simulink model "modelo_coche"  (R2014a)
settings: Solver=ode23t  StartTime=0.0  StopTime=10.0  MaxStep=0.2  RelTol=1e-3
undefined symbols (not defined in the file): inertiaLateral
libraries: nesl_utility x18, fl_lib x18, sdl_lib x10, simulink x1

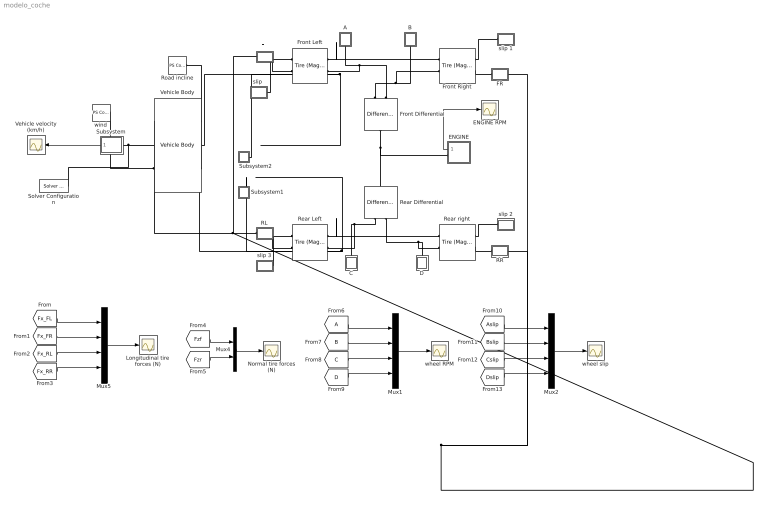
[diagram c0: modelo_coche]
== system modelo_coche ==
  A : Subsystem
  B : Subsystem
  C : Subsystem
  D : Subsystem
  ENGINE : Subsystem
  ENGINE RPM : Scope
  FL : Subsystem
  FR : Subsystem
  From6 : From  TagVisibility=global
  Front Differential : sdl_lib/Gears/Differential  driveshaft_location=2  cd_ratio=4  friction_model=1  efficiency=[ 0.85 0.92 ]  mu_visc=[ 0 0 ] N*m/(rad/s)  w_thr=[ 0.01 0.01 ] rad/s
  Front Left : sdl_lib/Tires & Vehicles/Tire (Magic Formula)  parameterization=1  F_z1=3e+3 N  F_x1=3.5e+3 N  kappa1=10  B_m=10  C_m=1.9  D_m=1  E_m=0.97  fz0=4e+3 N  p_Cx=1.685  p_Dx=[ 1.21 -0.037 ]  p_Ex=[ 0.344 0.095 -0.02 0 ]  p_Kx=[ 21.51 -0.163 0.245 ]  p_Hx=[ -0.002 0.002 ]  p_Vx=[ 0 0 ]  v_tr_thr=0.1 m/s  r_e=0.3 m  model_compliance=1  stiffness=tireStiffness N/m  damping=tireDamping N/(m/s)  model_inertia=1  inertia=inertiaLateral/2 kg*m^2  initial_velocity=0 rpm  model_resistance=1  resistance_model=1  coeff=0.015  p_tire=250e3 Pa  alpha=-0.003  beta=0.97  coeff_a=84e-4  coeff_b=6.2e-4 s/m  coeff_c=1.6e-4 s^2/m^2  v_thr=1e-3 m/s
  Front Right : sdl_lib/Tires & Vehicles/Tire (Magic Formula)  parameterization=1  F_z1=3e+3 N  F_x1=3.5e+3 N  kappa1=10  B_m=10  C_m=1.9  D_m=1  E_m=0.97  fz0=4e+3 N  p_Cx=1.685  p_Dx=[ 1.21 -0.037 ]  p_Ex=[ 0.344 0.095 -0.02 0 ]  p_Kx=[ 21.51 -0.163 0.245 ]  p_Hx=[ -0.002 0.002 ]  p_Vx=[ 0 0 ]  v_tr_thr=0.1 m/s  r_e=0.3 m  model_compliance=1  stiffness=tireStiffness N/m  damping=tireDamping N/(m/s)  model_inertia=1  inertia=inertiaLateral/2 kg*m^2  initial_velocity=0 rpm  model_resistance=1  resistance_model=1  coeff=0.015  p_tire=250e3 Pa  alpha=-0.003  beta=0.97  coeff_a=84e-4  coeff_b=6.2e-4 s/m  coeff_c=1.6e-4 s^2/m^2  v_thr=1e-3 m/s
  Longitudinal tire forces (N) : Scope
  Mux1 : Mux
  Mux2 : Mux
  Mux4 : Mux  Inputs=2
  Mux5 : Mux
  Normal tire forces (N) : Scope
  RL : Subsystem
  RR : Subsystem
  Rear Differential : sdl_lib/Gears/Differential  driveshaft_location=2  cd_ratio=4  friction_model=1  efficiency=[ 0.85 0.92 ]  mu_visc=[ 0 0 ] N*m/(rad/s)  w_thr=[ 0.01 0.01 ] rad/s
  Rear Left : sdl_lib/Tires & Vehicles/Tire (Magic Formula)  parameterization=1  F_z1=3e+3 N  F_x1=3.5e+3 N  kappa1=10  B_m=10  C_m=1.9  D_m=1  E_m=0.97  fz0=4e+3 N  p_Cx=1.685  p_Dx=[ 1.21 -0.037 ]  p_Ex=[ 0.344 0.095 -0.02 0 ]  p_Kx=[ 21.51 -0.163 0.245 ]  p_Hx=[ -0.002 0.002 ]  p_Vx=[ 0 0 ]  v_tr_thr=0.1 m/s  r_e=0.3 m  model_compliance=1  stiffness=tireStiffness N/m  damping=tireDamping N/(m/s)  model_inertia=1  inertia=inertiaLateral/2 kg*m^2  initial_velocity=0 rpm  model_resistance=1  resistance_model=1  coeff=0.015  p_tire=250e3 Pa  alpha=-0.003  beta=0.97  coeff_a=84e-4  coeff_b=6.2e-4 s/m  coeff_c=1.6e-4 s^2/m^2  v_thr=1e-3 m/s
  Rear right : sdl_lib/Tires & Vehicles/Tire (Magic Formula)  parameterization=1  F_z1=3e+3 N  F_x1=3.5e+3 N  kappa1=10  B_m=10  C_m=1.9  D_m=1  E_m=0.97  fz0=4e+3 N  p_Cx=1.685  p_Dx=[ 1.21 -0.037 ]  p_Ex=[ 0.344 0.095 -0.02 0 ]  p_Kx=[ 21.51 -0.163 0.245 ]  p_Hx=[ -0.002 0.002 ]  p_Vx=[ 0 0 ]  v_tr_thr=0.1 m/s  r_e=0.3 m  model_compliance=1  stiffness=tireStiffness N/m  damping=tireDamping N/(m/s)  model_inertia=1  inertia=inertiaLateral/2 kg*m^2  initial_velocity=0 rpm  model_resistance=1  resistance_model=1  coeff=0.015  p_tire=250e3 Pa  alpha=-0.003  beta=0.97  coeff_a=84e-4  coeff_b=6.2e-4 s/m  coeff_c=1.6e-4 s^2/m^2  v_thr=1e-3 m/s
  Road incline : fl_lib/Physical Signals/Sources/PS Constant  constant=0
  Solver Configuration : nesl_utility/Solver Configuration  PhysicalDomain=network_engine_domain  SubClassName=solver  LeftPortType=input  RightPortType=generic  Accelerate=off  Tones=[]  Harmonics=[]  SimulateNoise=off  Profile=off  UseLocalSampling=off  EnableSwitchedLinearOptims=on  FrequencyDomain=off  UseCCode=off  RelTol=0.001  AbsTol=1e-06  MinStep=1e-09  ToWorkspace=off  DoDC=off  ResidualTolerance=1e-9  UseLocalSolver=off  LocalSolverChoice=NE_BACKWARD_EULER_ADVANCER  LocalSolverSampleTime=0.1  DoFixedCost=off  MaxNonlinIter=3  MaxModeIter=2  LinearAlgebra=Sparse  DelaysMemoryBudget=1024  AutomaticFiltering=on  FilteringTimeConstant=0.001
  Subsystem : Subsystem
  Subsystem1 : Subsystem
  Subsystem2 : Subsystem
  Vehicle velocity (km/h) : Scope
  Vehicle Body : sdl_lib/Tires & Vehicles/Vehicle Body  mass=1500 kg  n_w=2  x_f=1.4 m  x_r=1.6 m  y_c=0.5 m  area=3 m^2  Cd=0.4  v0=0 m/s  g=9.81 m/s^2  rho=1.18 kg/m^3
  "slip " : Subsystem
  slip 1 : Subsystem
  slip 2 : Subsystem
  slip 3 : Subsystem
  wheel RPM : Scope
  wheel slip : Scope
  wind : fl_lib/Physical Signals/Sources/PS Constant  constant=0
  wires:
  Subsystem/1(km/h) -> Vehicle velocity (km/h)/1
  ENGINE/1(rpm) -> ENGINE RPM/1
  Mux5/1 -> Longitudinal tire forces (N)/1
  [Fx_FL] -> Mux5/1
  [Fx_FR] -> Mux5/2
  [Fx_RL] -> Mux5/3
  [Fx_RR] -> Mux5/4
  [Fzf] -> Mux4/1
  [Fzr] -> Mux4/2
  Mux4/1 -> Normal tire forces (N)/1
  Mux1/1 -> wheel RPM/1
  From6/1 -> Mux1/1
  [B] -> Mux1/2
  [C] -> Mux1/3
  [D] -> Mux1/4
  Mux2/1 -> wheel slip/1
  [Aslip] -> Mux2/1
  [Bslip] -> Mux2/2
  [Cslip] -> Mux2/3
  [Dslip] -> Mux2/4
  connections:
  Front Differential/RConn2 -- A/RConn1 -- Front Left/LConn2
  Front Differential/RConn1 -- B/RConn1 -- Front Right/LConn2
  Front Differential/LConn1 -- Rear Differential/LConn1 -- ENGINE/RConn1
  Rear Differential/RConn1 -- C/RConn1 -- Rear Left/LConn2
  Rear Differential/RConn2 -- D/RConn1 -- Rear right/LConn2
  Front Right/RConn2 -- FR/LConn1
  Rear right/RConn2 -- RR/LConn1
  RL/LConn1 -- Rear Left/RConn2
  FL/LConn1 -- Front Left/RConn2
  Front Left/LConn1 -- Subsystem2/LConn1 -- Vehicle Body/RConn2 -- Front Right/LConn1
  Rear Left/LConn1 -- Subsystem1/LConn1 -- Vehicle Body/RConn1 -- Rear right/LConn1
  "slip "/LConn1 -- Front Left/RConn1
  Front Right/RConn1 -- slip 1/LConn1
  Rear right/RConn1 -- slip 2/LConn1
  slip 3/LConn1 -- Rear Left/RConn1
  RL/RConn1 -- FR/RConn1 -- RR/RConn1 -- FL/RConn1 -- Vehicle Body/LConn1
  wind/RConn1 -- Vehicle Body/LConn3
  Road incline/RConn1 -- Vehicle Body/RConn3
  Subsystem/LConn1 -- Vehicle Body/LConn2 -- Solver Configuration/RConn1

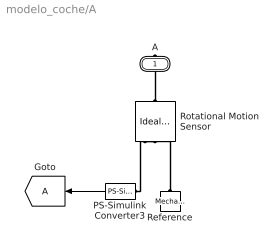
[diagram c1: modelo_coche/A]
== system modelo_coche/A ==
  Goto : Goto  TagVisibility=global
  PS-Simulink Converter3 : nesl_utility/PS-Simulink Converter  PhysicalDomain=network_engine_domain  SubClassName=ps_output  LeftPortType=input  RightPortType=output  PseudoPeriodic=off  Frequencies=[]  Unit=rpm  AffineConversion=off
  Reference : fl_lib/Mechanical/Rotational Elements/Mechanical Rotational Reference
  Rotational Motion Sensor : fl_lib/Mechanical/Mechanical Sensors/Ideal Rotational Motion Sensor  offset=0 rad
  A : PMIOPort  Port=1  Side=Right
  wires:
  PS-Simulink Converter3/1 -> Goto/1
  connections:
  Reference/LConn1 -- Rotational Motion Sensor/RConn1
  Rotational Motion Sensor/LConn1 -- A/RConn1
  PS-Simulink Converter3/LConn1 -- Rotational Motion Sensor/RConn2

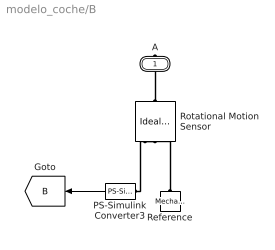
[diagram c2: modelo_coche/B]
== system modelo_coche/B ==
  PS-Simulink Converter3 : nesl_utility/PS-Simulink Converter  PhysicalDomain=network_engine_domain  SubClassName=ps_output  LeftPortType=input  RightPortType=output  PseudoPeriodic=off  Frequencies=[]  Unit=rpm  AffineConversion=off
  Reference : fl_lib/Mechanical/Rotational Elements/Mechanical Rotational Reference
  Rotational Motion Sensor : fl_lib/Mechanical/Mechanical Sensors/Ideal Rotational Motion Sensor  offset=0 rad
  A : PMIOPort  Port=1  Side=Right
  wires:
  PS-Simulink Converter3/1 -> [B]
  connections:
  PS-Simulink Converter3/LConn1 -- Rotational Motion Sensor/RConn2
  Rotational Motion Sensor/LConn1 -- A/RConn1
  Reference/LConn1 -- Rotational Motion Sensor/RConn1

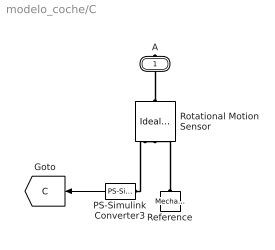
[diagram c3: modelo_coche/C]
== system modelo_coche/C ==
  PS-Simulink Converter3 : nesl_utility/PS-Simulink Converter  PhysicalDomain=network_engine_domain  SubClassName=ps_output  LeftPortType=input  RightPortType=output  PseudoPeriodic=off  Frequencies=[]  Unit=rpm  AffineConversion=off
  Reference : fl_lib/Mechanical/Rotational Elements/Mechanical Rotational Reference
  Rotational Motion Sensor : fl_lib/Mechanical/Mechanical Sensors/Ideal Rotational Motion Sensor  offset=0 rad
  A : PMIOPort  Port=1  Side=Right
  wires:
  PS-Simulink Converter3/1 -> [C]
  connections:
  PS-Simulink Converter3/LConn1 -- Rotational Motion Sensor/RConn2
  Rotational Motion Sensor/LConn1 -- A/RConn1
  Reference/LConn1 -- Rotational Motion Sensor/RConn1

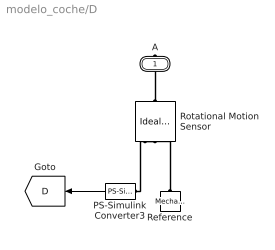
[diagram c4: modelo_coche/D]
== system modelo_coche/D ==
  PS-Simulink Converter3 : nesl_utility/PS-Simulink Converter  PhysicalDomain=network_engine_domain  SubClassName=ps_output  LeftPortType=input  RightPortType=output  PseudoPeriodic=off  Frequencies=[]  Unit=rpm  AffineConversion=off
  Reference : fl_lib/Mechanical/Rotational Elements/Mechanical Rotational Reference
  Rotational Motion Sensor : fl_lib/Mechanical/Mechanical Sensors/Ideal Rotational Motion Sensor  offset=0 rad
  A : PMIOPort  Port=1  Side=Right
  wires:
  PS-Simulink Converter3/1 -> [D]
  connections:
  Reference/LConn1 -- Rotational Motion Sensor/RConn1
  Rotational Motion Sensor/LConn1 -- A/RConn1
  PS-Simulink Converter3/LConn1 -- Rotational Motion Sensor/RConn2

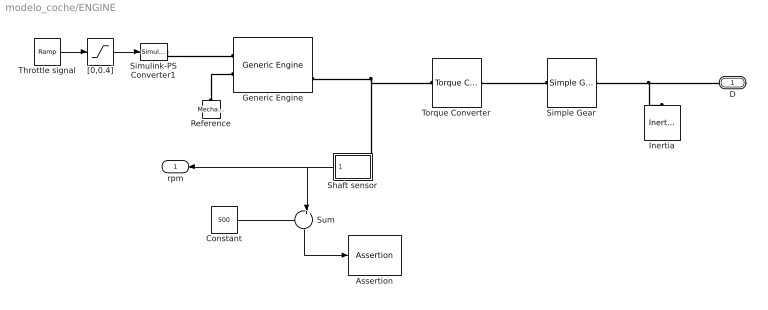
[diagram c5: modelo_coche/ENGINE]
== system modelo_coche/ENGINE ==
  Assertion : Assertion
  Constant : Constant  Value=500
  Generic Engine : sdl_lib/Engines/Generic Engine  model_parameterization=1  engine_type=1  P_max=1.5e+5 W  w_P_max=4.5e+3 rpm  w_max=6e+3 rpm  w_min=500 rpm  w_tab=[ 500 1000 2e+3 3e+3 4e+3 5e+3 6e+3 7e+3 ] rpm  trq_tab=[ 380 380 380 380 350 280 200 80 ] N*m  pwr_tab=[ 2e+4 4e+4 7.8e+4 1.2e+5 1.45e+5 1.48e+5 1.25e+5 6e+4 ] W  interp_method=1  model_inertia=0  inertia=1 kg*m^2  initial_velocity=800 rpm  model_time_constant=0  time_constant=0.2 s  T0=0  w_thr=100 rpm  idle_speed=0  idle_speed_reference=1000 rpm  tau_controller=1 s  idle_w_thr=1 rpm  fc_model=1  fc_per_rev=25 mg/rev  displaced_volume=400 cm^3  rev_per_cycle=2  fc_w_tab=[ 1000 2e+3 3e+3 4e+3 5e+3 6e+3 ] rpm  fc_trq_tab=[ 0 80 160 200 240 320 360 400 ] N*m  fc_tab=[ 0.5 0.9 1.4 1.6 1.9 2.7 3.4 4.4; 1 1.7 2.7 3.1 3.6 5 6 7.4; 1.4 2.7 4 4.8 5.6 7.5 8.5 10.5; 2 3.6 5.8 6.7 8 10.4 11.7 13.3; 2.5 4.8 7.9 9.4 10.8 14 16.2 18.6; 3.1 6 10.3 11.9 13.8 18.4 22 26.5 ] g/s  bmep_tab=[ 0 250 500 625 750 1000 1.15e+3 1.25e+3 ] kPa  bsfc_tab=[ 410 380 300 280 270 290 320 380; 410 370 290 270 260 270 285 320; 415 380 290 275 265 270 270 300; 420 390 310 290 285 280 280 285; 430 410 340 320 310 300 310 320; 450 430 370 340 330 330 350 380 ] g/hr/kW  fc_interp_method=1
  Inertia : fl_lib/Mechanical/Rotational Elements/Inertia  inertia=0.01 kg*m^2  w_specify=off  w_priority=High  w=0 rad/s  t_specify=off  t_priority=High  t=0 N*m
  Reference : fl_lib/Mechanical/Rotational Elements/Mechanical Rotational Reference
  Shaft sensor : Subsystem
  Simple Gear : sdl_lib/Gears/Simple Gear  ratio=2  rotation_direction=2  friction_model=1  T_noload=0.1 N*m  T_nom=5 N*m  efficiency_nom=0.8  efficiency=0.8  mu_visc=[ 0 0 ] N*m/(rad/s)  w_thr=0.01 rad/s
  Simulink-PS Converter1 : nesl_utility/Simulink-PS Converter  PhysicalDomain=network_engine_domain  SubClassName=ps_input  LeftPortType=input  RightPortType=output  PseudoPeriodic=off  Frequencies=[]  NoiseDistribution=none  NoiseParameters=[]  Unit=1  AffineConversion=off  InputFiltering=off  SimscapeFilterOrder=1  InputFilterTimeConstant=.001  UdotUserProvided=0
  Sum : Sum  Inputs=-+|
  Throttle signal : simulink/Sources/Ramp  slope=0.9/2  start=0  X0=0.02
  Torque Converter : sdl_lib/Couplings & Drives/Torque Converter  n_vector=[0 0.50 0.60 0.70 0.80 0.87 0.92 0.94 0.96 0.97]  trq_vector=[2.2320 1.5462 1.4058 1.2746 1.1528 1.0732 1.0192 0.9983 0.9983 0.9983]  cf_vector_parameterization=1  cf_vector_reference_speed=1  cf_vector=[12.2938 12.8588 13.1452 13.6285 14.6163 16.2675 19.3503 22.1046 29.9986 50.00] (rad/s)/(N*m)^0.5  cf_vector_sq=1e-3*[ 6.616 6.048 5.787 5.384 4.681 3.779 2.671 2.047 1.111 0.400] N*m/(rad/s)^2  interp_method=1  extrap_method=1  model_lag=0  tau=0.02 s  initial_trq_ratio=0
  "[0,0.4]" : Saturate  UpperLimit=0.4  LowerLimit=0
  D : PMIOPort  Port=1  Side=Right
  rpm : Outport
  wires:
  "[0,0.4]"/1 -> Simulink-PS Converter1/1
  Throttle signal/1 -> "[0,0.4]"/1
  Constant/1 -> Sum/1
  Sum/1 -> Assertion/1
  Shaft sensor/1(rpm) -> rpm/1, Sum/2
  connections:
  Torque Converter/RConn1 -- Simple Gear/LConn1
  Simple Gear/RConn1 -- D/RConn1 -- Inertia/LConn1
  Simulink-PS Converter1/RConn1 -- Generic Engine/LConn1
  Reference/LConn1 -- Generic Engine/LConn2
  Generic Engine/RConn3 -- Shaft sensor/LConn1 -- Torque Converter/LConn1

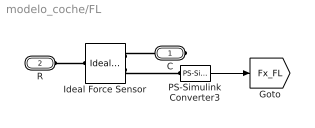
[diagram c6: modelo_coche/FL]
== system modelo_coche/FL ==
  Ideal Force Sensor : fl_lib/Mechanical/Mechanical Sensors/Ideal Force Sensor
  PS-Simulink Converter3 : nesl_utility/PS-Simulink Converter  PhysicalDomain=network_engine_domain  SubClassName=ps_output  LeftPortType=input  RightPortType=output  PseudoPeriodic=off  Frequencies=[]  Unit=N  AffineConversion=off
  C : PMIOPort  Port=1  Side=Right
  R : PMIOPort  Port=2  Side=Left
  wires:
  PS-Simulink Converter3/1 -> [Fx_FL]
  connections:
  Ideal Force Sensor/RConn2 -- PS-Simulink Converter3/LConn1
  Ideal Force Sensor/LConn1 -- R/RConn1
  Ideal Force Sensor/RConn1 -- C/RConn1

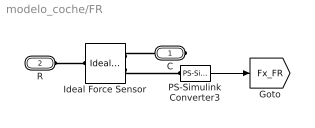
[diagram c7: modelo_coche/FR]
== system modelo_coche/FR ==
  Ideal Force Sensor : fl_lib/Mechanical/Mechanical Sensors/Ideal Force Sensor
  PS-Simulink Converter3 : nesl_utility/PS-Simulink Converter  PhysicalDomain=network_engine_domain  SubClassName=ps_output  LeftPortType=input  RightPortType=output  PseudoPeriodic=off  Frequencies=[]  Unit=N  AffineConversion=off
  C : PMIOPort  Port=1  Side=Right
  R : PMIOPort  Port=2  Side=Left
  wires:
  PS-Simulink Converter3/1 -> [Fx_FR]
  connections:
  Ideal Force Sensor/RConn2 -- PS-Simulink Converter3/LConn1
  Ideal Force Sensor/LConn1 -- R/RConn1
  Ideal Force Sensor/RConn1 -- C/RConn1

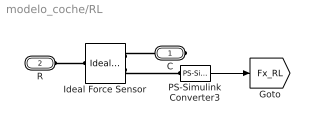
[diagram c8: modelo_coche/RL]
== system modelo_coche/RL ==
  Ideal Force Sensor : fl_lib/Mechanical/Mechanical Sensors/Ideal Force Sensor
  PS-Simulink Converter3 : nesl_utility/PS-Simulink Converter  PhysicalDomain=network_engine_domain  SubClassName=ps_output  LeftPortType=input  RightPortType=output  PseudoPeriodic=off  Frequencies=[]  Unit=N  AffineConversion=off
  C : PMIOPort  Port=1  Side=Right
  R : PMIOPort  Port=2  Side=Left
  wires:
  PS-Simulink Converter3/1 -> [Fx_RL]
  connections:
  Ideal Force Sensor/RConn1 -- C/RConn1
  Ideal Force Sensor/LConn1 -- R/RConn1
  Ideal Force Sensor/RConn2 -- PS-Simulink Converter3/LConn1

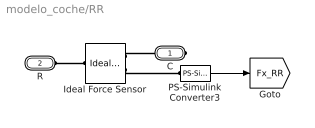
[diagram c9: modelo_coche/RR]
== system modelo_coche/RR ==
  Ideal Force Sensor : fl_lib/Mechanical/Mechanical Sensors/Ideal Force Sensor
  PS-Simulink Converter3 : nesl_utility/PS-Simulink Converter  PhysicalDomain=network_engine_domain  SubClassName=ps_output  LeftPortType=input  RightPortType=output  PseudoPeriodic=off  Frequencies=[]  Unit=N  AffineConversion=off
  C : PMIOPort  Port=1  Side=Right
  R : PMIOPort  Port=2  Side=Left
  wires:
  PS-Simulink Converter3/1 -> [Fx_RR]
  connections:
  Ideal Force Sensor/RConn2 -- PS-Simulink Converter3/LConn1
  Ideal Force Sensor/LConn1 -- R/RConn1
  Ideal Force Sensor/RConn1 -- C/RConn1

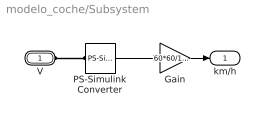
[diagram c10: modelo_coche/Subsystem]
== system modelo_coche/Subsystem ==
  Gain : Gain  Gain=60*60/1000
  PS-Simulink Converter : nesl_utility/PS-Simulink Converter  PhysicalDomain=network_engine_domain  SubClassName=ps_output  LeftPortType=input  RightPortType=output  PseudoPeriodic=off  Frequencies=[]  Unit=1  AffineConversion=off
  V : PMIOPort  Port=1  Side=Left
  km/h : Outport
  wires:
  PS-Simulink Converter/1 -> Gain/1
  Gain/1 -> km/h/1
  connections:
  PS-Simulink Converter/LConn1 -- V/RConn1

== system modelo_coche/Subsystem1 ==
  PS-Simulink Converter3 : nesl_utility/PS-Simulink Converter  PhysicalDomain=network_engine_domain  SubClassName=ps_output  LeftPortType=input  RightPortType=output  PseudoPeriodic=off  Frequencies=[]  Unit=N  AffineConversion=off
  f : PMIOPort  Port=1  Side=Left
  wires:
  PS-Simulink Converter3/1 -> [Fzr]
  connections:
  PS-Simulink Converter3/LConn1 -- f/RConn1

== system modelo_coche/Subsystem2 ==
  PS-Simulink Converter3 : nesl_utility/PS-Simulink Converter  PhysicalDomain=network_engine_domain  SubClassName=ps_output  LeftPortType=input  RightPortType=output  PseudoPeriodic=off  Frequencies=[]  Unit=N  AffineConversion=off
  f : PMIOPort  Port=1  Side=Left
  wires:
  PS-Simulink Converter3/1 -> [Fzf]
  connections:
  PS-Simulink Converter3/LConn1 -- f/RConn1

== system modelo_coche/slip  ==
  PS-Simulink Converter3 : nesl_utility/PS-Simulink Converter  PhysicalDomain=network_engine_domain  SubClassName=ps_output  LeftPortType=input  RightPortType=output  PseudoPeriodic=off  Frequencies=[]  Unit=N  AffineConversion=off
  S : PMIOPort  Port=1  Side=Left
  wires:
  PS-Simulink Converter3/1 -> [Aslip]
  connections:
  PS-Simulink Converter3/LConn1 -- S/RConn1

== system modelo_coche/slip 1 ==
  PS-Simulink Converter3 : nesl_utility/PS-Simulink Converter  PhysicalDomain=network_engine_domain  SubClassName=ps_output  LeftPortType=input  RightPortType=output  PseudoPeriodic=off  Frequencies=[]  Unit=N  AffineConversion=off
  S : PMIOPort  Port=1  Side=Left
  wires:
  PS-Simulink Converter3/1 -> [Bslip]
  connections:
  PS-Simulink Converter3/LConn1 -- S/RConn1

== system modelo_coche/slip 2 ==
  PS-Simulink Converter3 : nesl_utility/PS-Simulink Converter  PhysicalDomain=network_engine_domain  SubClassName=ps_output  LeftPortType=input  RightPortType=output  PseudoPeriodic=off  Frequencies=[]  Unit=N  AffineConversion=off
  S : PMIOPort  Port=1  Side=Left
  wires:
  PS-Simulink Converter3/1 -> [Dslip]
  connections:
  PS-Simulink Converter3/LConn1 -- S/RConn1

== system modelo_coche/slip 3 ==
  PS-Simulink Converter3 : nesl_utility/PS-Simulink Converter  PhysicalDomain=network_engine_domain  SubClassName=ps_output  LeftPortType=input  RightPortType=output  PseudoPeriodic=off  Frequencies=[]  Unit=N  AffineConversion=off
  S : PMIOPort  Port=1  Side=Left
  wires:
  PS-Simulink Converter3/1 -> [Cslip]
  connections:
  PS-Simulink Converter3/LConn1 -- S/RConn1

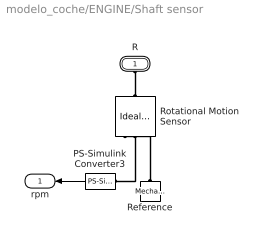
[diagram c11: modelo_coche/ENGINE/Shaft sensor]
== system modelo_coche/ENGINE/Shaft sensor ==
  PS-Simulink Converter3 : nesl_utility/PS-Simulink Converter  PhysicalDomain=network_engine_domain  SubClassName=ps_output  LeftPortType=input  RightPortType=output  PseudoPeriodic=off  Frequencies=[]  Unit=rpm  AffineConversion=off
  Reference : fl_lib/Mechanical/Rotational Elements/Mechanical Rotational Reference
  Rotational Motion Sensor : fl_lib/Mechanical/Mechanical Sensors/Ideal Rotational Motion Sensor  offset=0 rad
  R : PMIOPort  Port=1  Side=Left
  rpm : Outport
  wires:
  PS-Simulink Converter3/1 -> rpm/1
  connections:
  R/RConn1 -- Rotational Motion Sensor/LConn1
  Reference/LConn1 -- Rotational Motion Sensor/RConn1
  Rotational Motion Sensor/RConn2 -- PS-Simulink Converter3/LConn1
